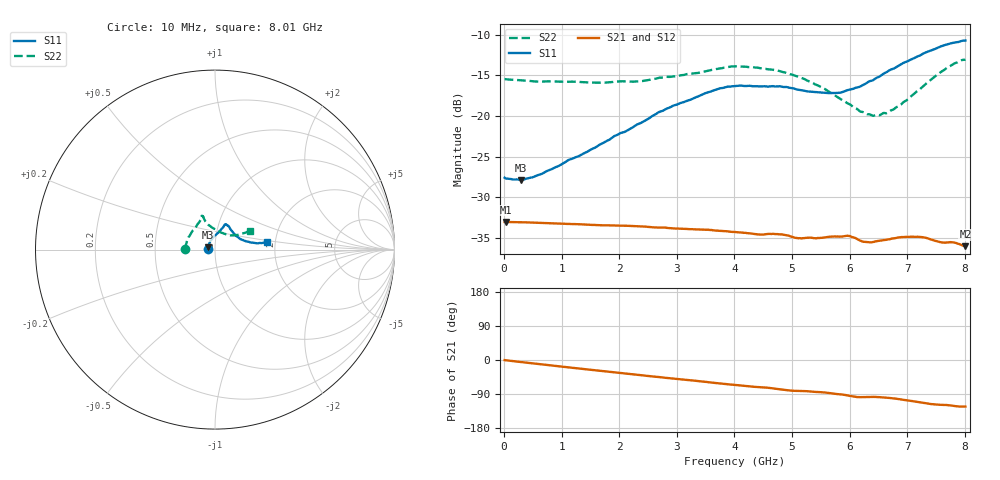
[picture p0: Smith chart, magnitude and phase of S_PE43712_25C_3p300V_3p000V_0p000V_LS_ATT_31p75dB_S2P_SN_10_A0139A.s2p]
! DEVICE ID: PE43712
! File Path: z:\PE43713\PE43713_CHAR_NOM_04292014\AMB\3p300\LS_ATT_31p75dB\PE43713_AMB_3p300V_3p000V_0p000V_LS_ATT_31p75dB_S2P_SN_10_A0139A.s2p
! Serial: 10
! Lot: A0139A
! Temp: 25C
! VDD: 3.300
! VSS: 0.000
! Control_Hi: 3.000
! Control_Lo: 0.000
! Attenuation Step: 31.75dB
! Port 1: RF1
! Port 2: RF2
! ThroughPath:1-2
! IDD: 0.000145913
! ISS: -6.48e-008
#  Hz  S  RI  R  50
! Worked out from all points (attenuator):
!   801 points, 10 MHz to 8.01 GHz, reference 50 ohm
!   highest |S21| = -33.04 dB at 30 MHz (marker M1); lowest = -36.0 dB at 8.01 GHz (marker M2)
!   lowest |S11| = -27.9 dB at 290 MHz (marker M3), VSWR 1.08, Z = 46.3 + j1.23 ohm
!   |S11| at or under -10 dB: start of sweep to end of sweep
!   |S22| runs from -20.0 to -13.0 dB; largest |S21 - S12| = 9.9e-05
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1e7  -0.0417 0.000882  0.0223 -9.9e-05  0.0223 -7.33e-05  -0.1689 0.00113
3e7  -0.0412 0.0022  0.0223 -0.000226  0.0223 -0.000228  -0.1684 0.0028
2.9e8  -0.0381 0.0133  0.0221 -0.00206  0.0221 -0.00206  -0.1648 0.0175
6.5e8  -0.0338 0.0281  0.0215 -0.00443  0.0215 -0.00443  -0.1587 0.0371
1.35e9  -0.021 0.054  0.0198 -0.00853  0.0198 -0.00853  -0.1449 0.0719
2.31e9  0.0103 0.0881  0.0163 -0.0132  0.0163 -0.0132  -0.1119 0.1187
2.68e9  0.025 0.1024  0.0146 -0.0145  0.0146 -0.0145  -0.0971 0.1417
3.5e9  0.0484 0.1298  0.0107 -0.0169  0.0106 -0.0169  -0.0762 0.1724
4.01e9  0.0582 0.1416  0.00792 -0.0176  0.00789 -0.0176  -0.0747 0.1881
4.44e9  0.0638 0.1382  0.00588 -0.0177  0.00588 -0.0177  -0.0674 0.1853
4.76e9  0.0722 0.1345  0.00429 -0.0182  0.00432 -0.0182  -0.0636 0.1792
5.09e9  0.0821 0.1201  0.00265 -0.0175  0.00268 -0.0175  -0.0572 0.166
5.35e9  0.0911 0.1073  0.00197 -0.0177  0.00191 -0.0177  -0.051 0.1523
5.83e9  0.115 0.0784  -0.000155 -0.0181  -0.000157 -0.0181  -0.0209 0.1261
5.98e9  0.1263 0.0709  -0.0013 -0.0182  -0.00123 -0.0183  -0.00835 0.1187
6.29e9  0.1493 0.0551  -0.00224 -0.0166  -0.0022 -0.0166  0.0225 0.1006
6.42e9  0.1595 0.0507  -0.00218 -0.0167  -0.00215 -0.0166  0.0368 0.0934
6.68e9  0.1853 0.0434  -0.00299 -0.0172  -0.003 -0.0171  0.0662 0.0832
6.87e9  0.2017 0.039  -0.00419 -0.0174  -0.00417 -0.0174  0.0844 0.0797
7.22e9  0.233 0.0354  -0.00665 -0.0167  -0.00661 -0.0167  0.1215 0.0814
7.7e9  0.274 0.0391  -0.00809 -0.0146  -0.00804 -0.0145  0.1746 0.0966
8.01e9  0.2887 0.0432  -0.00855 -0.0133  -0.00849 -0.0133  0.1961 0.1057
